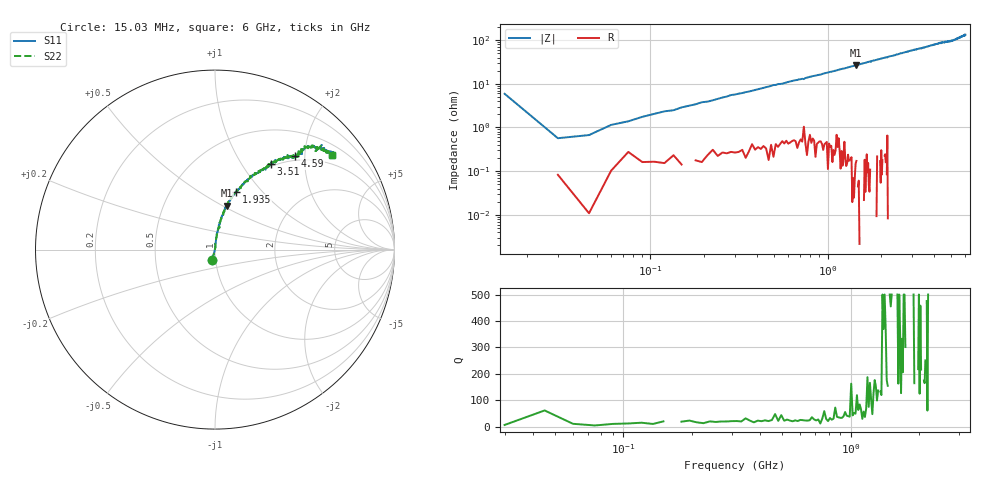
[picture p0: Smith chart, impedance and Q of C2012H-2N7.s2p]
!	Network	Analyzer	HP8753E.07.74:	Oct	30	2002	Serial	No.	JP38451487
!	Hewlett-Packard
!	28	Aug	2009	9:36:41
!	Frequency	S11	S21	S12	S22
#	HZ	S	RI	R	50
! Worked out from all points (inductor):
!   400 points, 15.03 MHz to 6 GHz, reference 50 ohm
!   read as one part in series: L = 2.88 nH near 45.03 MHz
!   highest Q = 370 at 1.44 GHz (marker M1), where L = 2.9 nH
!   S11 on the Smith chart (normalised r, x): 15.03 MHz: 0.96, -0.11; 1.935 GHz: 1.00, +0.73; 3.51 GHz: 0.96, +1.36; 4.59 GHz: 0.92, +1.80; 6 GHz: 0.73, +2.64
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1.502992e7  -0.0152 -0.0576  1.02 0.0576  1.02 0.0576  -0.0152 -0.0576
3.002985e7  0.000715 0.00561  0.999 -0.00561  0.999 -0.00561  0.000715 0.00561
4.502978e7  0.000307 0.0067  1 -0.0067  1 -0.0067  0.000307 0.0067
6.00297e7  0.00131 0.0114  0.999 -0.0114  0.999 -0.0114  0.00131 0.0114
9.002955e7  0.00183 0.0174  0.998 -0.0174  0.998 -0.0174  0.00183 0.0174
1.200294e8  0.00214 0.0233  0.998 -0.0233  0.998 -0.0233  0.00214 0.0233
1.95029e8  0.00306 0.0376  0.997 -0.0376  0.997 -0.0376  0.00306 0.0376
2.850286e8  0.00555 0.0548  0.994 -0.0548  0.994 -0.0548  0.00555 0.0548
4.950275e8  0.0106 0.0926  0.989 -0.0926  0.989 -0.0926  0.0106 0.0926
1.020025e9  0.0366 0.177  0.963 -0.177  0.963 -0.177  0.0366 0.177
1.440023e9  0.0655 0.245  0.934 -0.245  0.934 -0.245  0.0655 0.245
1.93502e9  0.118 0.323  0.882 -0.323  0.882 -0.323  0.118 0.323
2.01002e9  0.127 0.329  0.873 -0.329  0.873 -0.329  0.127 0.329
3.015015e9  0.253 0.443  0.747 -0.443  0.747 -0.443  0.253 0.443
3.510012e9  0.312 0.478  0.688 -0.478  0.688 -0.478  0.312 0.478
4.00501e9  0.385 0.516  0.615 -0.516  0.615 -0.516  0.385 0.516
4.590007e9  0.447 0.52  0.553 -0.52  0.553 -0.52  0.447 0.52
5.010005e9  0.479 0.545  0.521 -0.545  0.521 -0.545  0.479 0.545
5.415003e9  0.544 0.58  0.456 -0.58  0.456 -0.58  0.544 0.58
5.535002e9  0.56 0.549  0.44 -0.549  0.44 -0.549  0.56 0.549
5.565002e9  0.595 0.583  0.405 -0.583  0.405 -0.583  0.595 0.583
6e9  0.653 0.529  0.347 -0.529  0.347 -0.529  0.653 0.529
